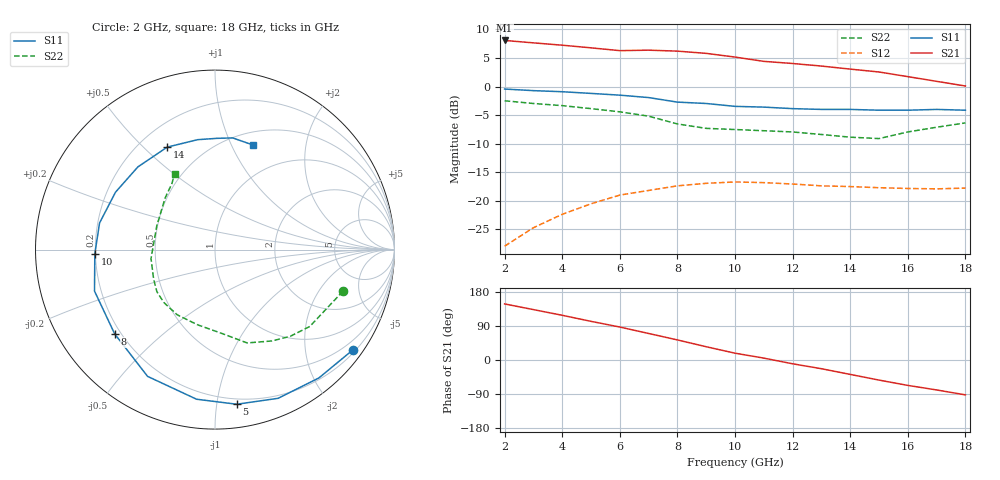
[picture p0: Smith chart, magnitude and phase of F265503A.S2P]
!ATF-26550
!S-PARAMETERS at Vds=3V  Id=`0mA.  LAST UPDATED 07-22-92
# ghz s ma r 50
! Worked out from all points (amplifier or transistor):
!   17 points, 2 GHz to 18 GHz, reference 50 ohm
!   highest |S21| = 8.1 dB at 2 GHz (marker M1)
!   |S21| within 3 dB of that: start of sweep to 10.12 GHz
!   unconditionally stable (mu >= 1): 11.04 GHz to end of sweep
!   at 4 GHz: K = 0.41, MSG = 14.8 dB, |S12| = -22.4 dB
!   at 10 GHz: K = 0.90, MSG = 10.9 dB, |S12| = -16.7 dB
!   at 18 GHz: K = 1.59, MAG = 4.4 dB, |S12| = -17.8 dB
!   S11 on the Smith chart (normalised r, x): 2 GHz: 0.27, -3.06; 5 GHz: 0.16, -1.14; 8 GHz: 0.18, -0.35; 10 GHz: 0.20, -0.02; 14 GHz: 0.31, +0.59; 18 GHz: 0.64, +1.21
2  0.95 -36.0  2.53 148.0  0.04 64.0  0.75 -18.0
3  0.92 -51.0  2.41 133.0  0.058 55.0  0.71 -26.0
4  0.9 -67.0  2.3 118.0  0.076 43.0  0.68 -39.0
5  0.87 -82.0  2.18 102.0  0.094 34.0  0.64 -49.0
6  0.84 -97.0  2.06 87.0  0.112 24.0  0.6 -58.0
7  0.8 -118.0  2.08 70.0  0.123 7.0  0.55 -71.0
8  0.73 -140.0  2.04 53.0  0.135 -5.0  0.47 -85.0
9  0.71 -161.0  1.95 35.0  0.142 -17.0  0.43 -103.0
10  0.67 -178.0  1.81 18.0  0.146 -27.0  0.42 -120.0
11  0.66 167.0  1.66 5.0  0.144 -39.0  0.41 -134.0
12  0.64 150.0  1.59 -10.0  0.14 -49.0  0.4 -144.0
13  0.63 133.0  1.51 -23.0  0.135 -59.0  0.38 -154.0
14  0.63 115.0  1.42 -38.0  0.133 -66.0  0.36 -172.0
15  0.62 99.0  1.34 -53.0  0.13 -74.0  0.35 158.0
16  0.62 89.0  1.22 -67.0  0.128 -88.0  0.4 134.0
17  0.63 81.0  1.11 -79.0  0.127 -91.0  0.44 123.0
18  0.62 70.0  1.01 -92.0  0.129 -94.0  0.48 118.0
